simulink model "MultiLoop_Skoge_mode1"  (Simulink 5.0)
settings: Solver=ode1  SolverMode=SingleTasking  StartTime=0.0  StopTime=100  FixedStep=Ts_base  MaxStep=Ts_base  MinStep=1e-6  RelTol=1e-6
PreLoadFcn:
  | Skoge_Mode1_Init
StopFcn:
  | teplot
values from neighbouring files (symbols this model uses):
  Ts_base = 0.0005    [Skoge_Mode1_Init.m]
  Ts_save = 0.01    [Skoge_Mode1_Init.m]
libraries: TElib x17, simulink x8

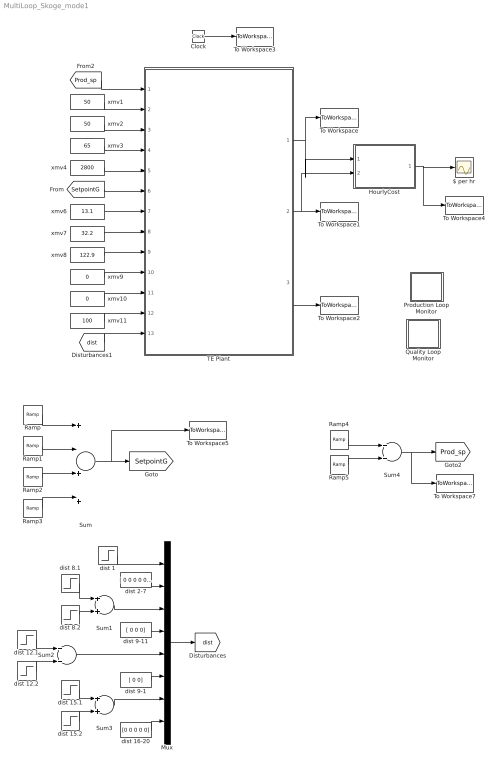
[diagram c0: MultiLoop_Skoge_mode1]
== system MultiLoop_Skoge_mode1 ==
  $ per hr : Scope
  Clock : Clock
  HourlyCost : Subsystem
  Mux : Mux  Inputs=8
  Production Loop Monitor : Subsystem
  Quality Loop Monitor : Subsystem
  Ramp : simulink/Sources/Ramp  slope=-1  start=35  X0=53.8
  Ramp1 : simulink/Sources/Ramp  slope=1  start=45  X0=0
  Ramp2 : simulink/Sources/Ramp  slope=1  start=50  X0=0
  Ramp3 : simulink/Sources/Ramp  slope=-1  start=60  X0=0
  Ramp4 : simulink/Sources/Ramp  slope=.25  start=80  X0=22.89
  Ramp5 : simulink/Sources/Ramp  slope=-.25  start=95  X0=0
  Sum : Sum  Inputs=+|+|+|+  ShowAdditionalParam=on
  Sum{1..4} (4 alike) : Sum
  TE Plant : Subsystem
  To Workspace : ToWorkspace  VariableName=simout  SampleTime=Ts_save  SaveFormat=Array
  To Workspace1 : ToWorkspace  VariableName=xmv  SampleTime=Ts_save  SaveFormat=Array
  To Workspace2 : ToWorkspace  VariableName=idv  SampleTime=Ts_save  SaveFormat=Array
  To Workspace3 : ToWorkspace  VariableName=tout  SampleTime=Ts_save  SaveFormat=Array
  To Workspace4 : ToWorkspace  VariableName=OpCost  SampleTime=Ts_save  SaveFormat=Array
  To Workspace5 : ToWorkspace  VariableName=molG_sp  SampleTime=Ts_save  SaveFormat=Array
  To Workspace7 : ToWorkspace  VariableName=Prod_sp  SampleTime=Ts_save  SaveFormat=Array
  dist 1 : Step  Time=22  Before=1  After=0  SampleTime=0
  dist 12.1 : Step  Time=65  SampleTime=0
  dist 12.2 : Step  Time=70  After=-1  SampleTime=0
  dist 15.1 : Step  Time=65  SampleTime=0
  dist 15.2 : Step  Time=70  After=-1  SampleTime=0
  dist 16-20 : Constant  Value=[0 0 0 0 0]
  dist 2-7 : Constant  Value=[ 0 0 0 0 0 0]
  dist 8.1 : Step  Time=70  SampleTime=0
  dist 8.2 : Step  Time=75  After=-1  SampleTime=0
  dist 9-1 : Constant  Value=[ 0 0]
  dist 9-11 : Constant  Value=[ 0 0 0]
  xmv1 : Constant  Value=50
  xmv10 : Constant  Value=0
  xmv11 : Constant  Value=100
  xmv2 : Constant  Value=50
  xmv3 : Constant  Value=65
  xmv4 : Constant  Value=2800
  xmv6 : Constant  Value=13.1
  xmv7 : Constant  Value=32.2
  xmv8 : Constant  Value=122.9
  xmv9 : Constant  Value=0
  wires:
  TE Plant/1(xmeas) -> To Workspace/1, HourlyCost/1(xmeas)
  xmv1/1 -> TE Plant/2(Strip Level Setpoint)
  xmv2/1 -> TE Plant/3(Sep Level Setpoint)
  xmv3/1 -> TE Plant/4(Reactor Level Setpoint)
  xmv4/1 -> TE Plant/5(Reactor Press Setpoint)
  xmv8/1 -> TE Plant/9(Reactor Temp Setpoint)
  xmv6/1 -> TE Plant/7(%C Setpoint)
  xmv7/1 -> TE Plant/8(Recycle Rate Setpt)
  TE Plant/2(xmv) -> To Workspace1/1, HourlyCost/2(xmv)
  TE Plant/3(idv) -> To Workspace2/1
  Clock/1 -> To Workspace3/1
  HourlyCost/1($ per hr) -> $ per hr/1, To Workspace4/1
  xmv9/1 -> TE Plant/10(Recycle Valve Position)
  xmv10/1 -> TE Plant/11(Steam Valve Position)
  xmv11/1 -> TE Plant/12(Agitator Setting)
  [dist] -> TE Plant/13(Disturbances)
  [SetpointG] -> TE Plant/6(Mole % G Setpoint)
  Ramp/1 -> Sum/1
  Ramp1/1 -> Sum/2
  Ramp2/1 -> Sum/3
  Ramp3/1 -> Sum/4
  Sum/1 -> [SetpointG], To Workspace5/1
  [Prod_sp] -> TE Plant/1(Production Setpoint)
  dist 1/1 -> Mux/1
  dist 2-7/1 -> Mux/2
  dist 8.1/1 -> Sum1/1
  dist 8.2/1 -> Sum1/2
  dist 12.1/1 -> Sum2/1
  dist 12.2/1 -> Sum2/2
  dist 15.1/1 -> Sum3/1
  dist 15.2/1 -> Sum3/2
  Sum1/1 -> Mux/3
  dist 9-11/1 -> Mux/4
  Sum2/1 -> Mux/5
  dist 9-1/1 -> Mux/6
  Sum3/1 -> Mux/7
  dist 16-20/1 -> Mux/8
  Mux/1 -> [dist]
  Ramp4/1 -> Sum4/1
  Ramp5/1 -> Sum4/2
  Sum4/1 -> [Prod_sp], To Workspace7/1

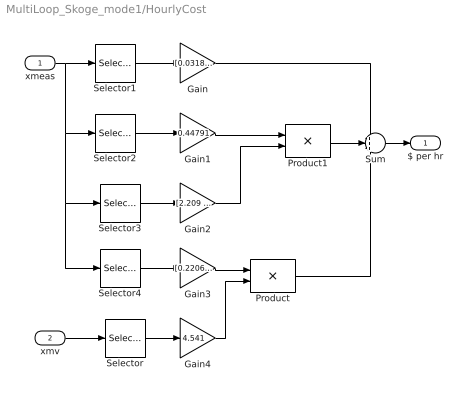
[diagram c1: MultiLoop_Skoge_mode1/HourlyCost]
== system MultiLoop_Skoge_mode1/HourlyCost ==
  xmeas : Inport  PortDimensions=41
  xmv : Inport  Port=2  PortDimensions=12
  Gain : Gain  Gain=[0.0318, 0.0536]  Multiplication=Matrix(K*u)
  Gain1 : Gain  Gain=0.44791
  Gain2 : Gain  Gain=[2.209 6.177 22.06 14.56 17.89 30.44 22.94]  Multiplication=Matrix(K*u)
  Gain3 : Gain  Gain=[0.2206 0.1456 0.1789]  Multiplication=Matrix(K*u)
  Gain4 : Gain  Gain=4.541
  Product : Product
  Product1 : Product
  Selector : Selector  Elements=8  InputPortWidth=12
  Selector1 : Selector  Elements=[19 20]  InputPortWidth=41
  Selector2 : Selector  Elements=[10]  InputPortWidth=41
  Selector3 : Selector  Elements=[29, 31:36]  InputPortWidth=41
  Selector4 : Selector  Elements=[37:39]  InputPortWidth=41
  Sum : Sum  Inputs=+++
  $ per hr : Outport
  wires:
  xmv/1 -> Selector/1
  xmeas/1 -> Selector1/1, Selector2/1, Selector3/1, Selector4/1
  Selector1/1 -> Gain/1
  Selector2/1 -> Gain1/1
  Selector3/1 -> Gain2/1
  Selector4/1 -> Gain3/1
  Selector/1 -> Gain4/1
  Gain3/1 -> Product/1
  Gain4/1 -> Product/2
  Sum/1 -> $ per hr/1
  Product/1 -> Sum/3
  Gain/1 -> Sum/1
  Product1/1 -> Sum/2
  Gain1/1 -> Product1/1
  Gain2/1 -> Product1/2

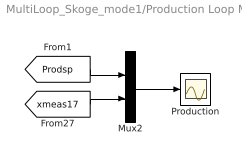
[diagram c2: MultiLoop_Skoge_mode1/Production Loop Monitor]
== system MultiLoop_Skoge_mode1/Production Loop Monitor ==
  Mux2 : Mux  Inputs=2
  Production : Scope
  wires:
  Mux2/1 -> Production/1
  [xmeas17] -> Mux2/2
  [Prodsp] -> Mux2/1

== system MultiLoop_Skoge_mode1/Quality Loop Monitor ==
  Mux2 : Mux  Inputs=2
  Quality : Scope
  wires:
  [PctGsp] -> Mux2/1
  [xmeas40] -> Mux2/2
  Mux2/1 -> Quality/1

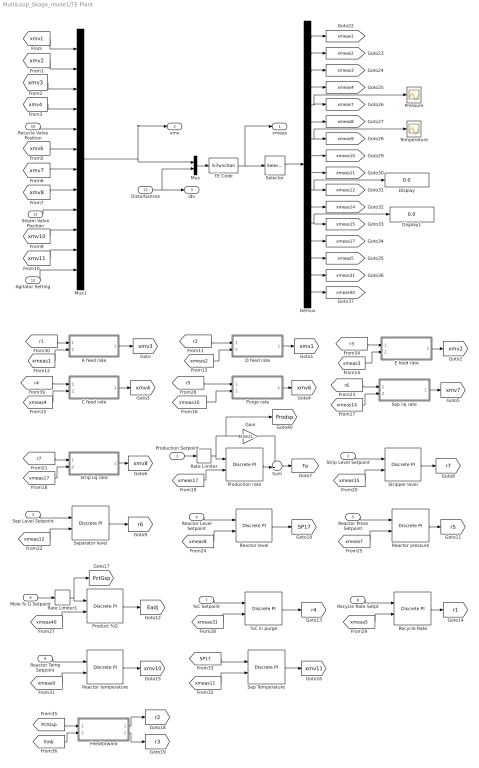
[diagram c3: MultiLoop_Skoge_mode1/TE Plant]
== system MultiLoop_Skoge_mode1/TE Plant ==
  Production Setpoint : Inport
  Strip Level Setpoint : Inport  Port=2
  Sep Level Setpoint : Inport  Port=3
  Reactor Level Setpoint : Inport  Port=4
  Reactor Press Setpoint : Inport  Port=5
  Mole % G Setpoint : Inport  Port=6
  %C Setpoint : Inport  Port=7
  Recycle Rate Setpt : Inport  Port=8
  Reactor Temp Setpoint : Inport  Port=9
  Recycle Valve Position : Inport  Port=10
  Steam Valve Position : Inport  Port=11
  Agitator Setting : Inport  Port=12
  Disturbances : Inport  Port=13
  %C in purge : TElib/Discrete PI  Kc=0.0009  Ti=562/60  Ts=Ts_base  x0=r4_0  Hi=200  Lo=0
  A feed rate : Subsystem
  C feed rate : Subsystem
  D feed rate : Subsystem
  Demux : Demux  Outputs=16
  Display : Display
  Display1 : Display
  E feed rate : Subsystem
  Feedforward : Subsystem
  Gain : Gain  Gain=100/22.89
  Mux : Mux  Inputs=2
  Mux1 : Mux  Inputs=12
  Pressure : Scope
  Product %G : TElib/Discrete PI  Kc=-0.032  Ti=100/60  Ts=Ts_base  x0=Eadj_0  Hi=inf  Lo=-inf
  Production rate : TElib/Discrete PI  Kc=3.2  Ti=120/60  Ts=Ts_base  x0=0  Hi=20  Lo=-20
  Purge rate : Subsystem
  Rate Limiter : RateLimiter  RisingSlewLimit=0.3*22.95/24  FallingSlewLimit=-0.3*22.95/24
  Rate Limiter1 : RateLimiter  RisingSlewLimit=50/24  FallingSlewLimit=-50/24
  Reactor level : TElib/Discrete PI  Kc=0.8  Ti=60/60  Ts=Ts_base  x0=SP17_0  Hi=120  Lo=0
  Reactor pressure : TElib/Discrete PI  Kc=-1e-4  Ti=20/60  Ts=Ts_base  x0=r5_0  Hi=100  Lo=0
  Reactor temperature : TElib/Discrete PI  Kc=-8  Ti=7.5/60  Ts=Ts_base  x0=xmv10_0  Hi=100  Lo=0
  Recycle Rate : TElib/Discrete PI  Kc=0.00125  Ti=120/60  Ts=Ts_base  x0=r1_0  Hi=200  Lo=0
  Selector : Selector  Elements=[1:4, 7:12, 14, 15, 17, 5, 31, 40]  InputPortWidth=41
  Sep Temperature : TElib/Discrete PI  Kc=-4  Ti=15/60  Ts=Ts_base  x0=xmv11_0  Hi=100  Lo=0
  Sep liq rate : Subsystem
  Separator level : TElib/Discrete PI  Kc=-1e-3  Ti=200/60  Ts=Ts_base  x0=r6_0  Hi=100  Lo=0
  Strip liq rate : Subsystem
  Stripper level : TElib/Discrete PI  Kc=-2e-4  Ti=200/60  Ts=Ts_base  x0=r7_0  Hi=100  Lo=0
  Sum : Sum  Inputs=++|
  TE Code : S-Function  FunctionName=temexd  Parameters=[]
  Temperature : Scope
  xmeas : Outport
  xmv : Outport  Port=2
  idv : Outport  Port=3
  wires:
  Mux/1 -> TE Code/1
  Disturbances/1 -> Mux/2, idv/1
  TE Code/1 -> xmeas/1, Selector/1
  [xmv1] -> Mux1/1
  [xmv2] -> Mux1/2
  [xmv3] -> Mux1/3
  [xmv4] -> Mux1/4
  Recycle Valve Position/1 -> Mux1/5
  [xmv6] -> Mux1/6
  [xmv7] -> Mux1/7
  [xmv8] -> Mux1/8
  Steam Valve Position/1 -> Mux1/9
  [xmv10] -> Mux1/10
  [xmv11] -> Mux1/11
  Agitator Setting/1 -> Mux1/12
  A feed rate/1(Valve %) -> [xmv3]
  [xmeas1] -> A feed rate/2(Measured Flow)
  D feed rate/1(Valve %) -> [xmv1]
  [xmeas2] -> D feed rate/2(Measured Flow)
  E feed rate/1(Valve %) -> [xmv2]
  [xmeas3] -> E feed rate/2(Measured Flow)
  C feed rate/1(Valve %) -> [xmv4]
  [xmeas4] -> C feed rate/2(Measured Flow)
  Purge rate/1(Valve %) -> [xmv6]
  [xmeas10] -> Purge rate/2(Measured Flow)
  Sep liq rate/1(Valve %) -> [xmv7]
  [xmeas14] -> Sep liq rate/2(Measured Flow)
  Strip liq rate/1(Valve %) -> [xmv8]
  [xmeas17] -> Strip liq rate/2(Measured Flow)
  [xmeas17] -> Production rate/2
  [xmeas15] -> Stripper level/2
  Strip Level Setpoint/1 -> Stripper level/1
  Stripper level/1 -> [r7]
  [r7] -> Strip liq rate/1(Ratio)
  [xmeas12] -> Separator level/2
  Sep Level Setpoint/1 -> Separator level/1
  Separator level/1 -> [r6]
  [r6] -> Sep liq rate/1(Ratio)
  [xmeas8] -> Reactor level/2
  Reactor Level Setpoint/1 -> Reactor level/1
  Reactor level/1 -> [SP17]
  [xmeas7] -> Reactor pressure/2
  Reactor Press Setpoint/1 -> Reactor pressure/1
  Reactor pressure/1 -> [r5]
  [r5] -> Purge rate/1(Ratio)
  [xmeas40] -> Product %G/2
  Product %G/1 -> [Eadj]
  [xmeas31] -> %C in purge/2
  %C Setpoint/1 -> %C in purge/1
  %C in purge/1 -> [r4]
  [xmeas5] -> Recycle Rate/2
  Recycle Rate Setpt/1 -> Recycle Rate/1
  Recycle Rate/1 -> [r1]
  [r1] -> A feed rate/1(Ratio)
  [xmeas9] -> Reactor temperature/2
  Reactor Temp Setpoint/1 -> Reactor temperature/1
  Reactor temperature/1 -> [xmv10]
  [xmeas11] -> Sep Temperature/2
  [SP17] -> Sep Temperature/1
  Sep Temperature/1 -> [xmv11]
  [r2] -> D feed rate/1(Ratio)
  [r3] -> E feed rate/1(Ratio)
  [PctGsp] -> Feedforward/1(Mole % G SP)
  [Eadj] -> Feedforward/2(Eadj)
  Feedforward/1(r2) -> [r2]
  Feedforward/2(r3) -> [r3]
  Mux1/1 -> Mux/1, xmv/1
  Selector/1 -> Demux/1
  Demux/1 -> [xmeas1]
  Demux/2 -> [xmeas2]
  Demux/3 -> [xmeas3]
  Demux/4 -> [xmeas4]
  Demux/5 -> [xmeas7], Pressure/1
  Demux/6 -> [xmeas8]
  Demux/7 -> [xmeas9], Temperature/1
  Demux/8 -> [xmeas10]
  Demux/9 -> [xmeas11]
  Demux/10 -> [xmeas12], Display/1
  Demux/11 -> [xmeas14]
  Demux/12 -> [xmeas15], Display1/1
  Demux/13 -> [xmeas17]
  Demux/14 -> [xmeas5]
  Demux/15 -> [xmeas31]
  Demux/16 -> [xmeas40]
  [r4] -> C feed rate/1(Ratio)
  Rate Limiter1/1 -> Product %G/1, [PctGsp]
  Mole % G Setpoint/1 -> Rate Limiter1/1
  Rate Limiter/1 -> Production rate/1, Gain/1, [Prodsp]
  Production Setpoint/1 -> Rate Limiter/1
  Sum/1 -> [Fp]
  Production rate/1 -> Sum/2
  Gain/1 -> Sum/1

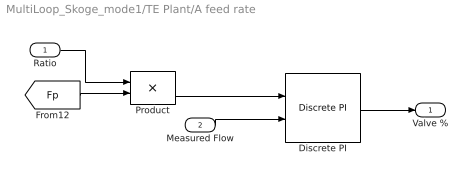
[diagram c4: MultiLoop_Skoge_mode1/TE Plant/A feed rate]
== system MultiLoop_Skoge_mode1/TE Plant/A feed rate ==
  Ratio : Inport
  Measured Flow : Inport  Port=2
  Discrete PI : TElib/Discrete PI  Kc=0.01  Ti=0.001/60  Ts=Ts_base  x0=xmv3_0  Hi=100  Lo=0
  Product : Product
  Valve % : Outport
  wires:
  Discrete PI/1 -> Valve %/1
  Ratio/1 -> Product/1
  [Fp] -> Product/2
  Measured Flow/1 -> Discrete PI/2
  Product/1 -> Discrete PI/1

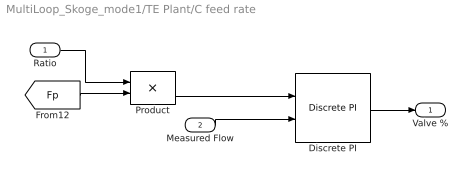
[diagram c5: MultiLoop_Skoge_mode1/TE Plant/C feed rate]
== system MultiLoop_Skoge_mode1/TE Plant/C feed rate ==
  Ratio : Inport
  Measured Flow : Inport  Port=2
  Discrete PI : TElib/Discrete PI  Kc=0.003  Ti=0.001/60  Ts=Ts_base  x0=xmv4_0  Hi=100  Lo=0
  Product : Product
  Valve % : Outport
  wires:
  Product/1 -> Discrete PI/1
  Measured Flow/1 -> Discrete PI/2
  [Fp] -> Product/2
  Ratio/1 -> Product/1
  Discrete PI/1 -> Valve %/1

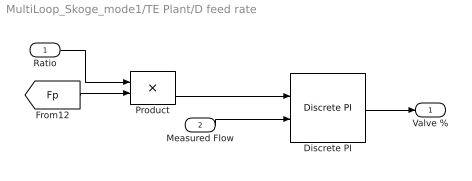
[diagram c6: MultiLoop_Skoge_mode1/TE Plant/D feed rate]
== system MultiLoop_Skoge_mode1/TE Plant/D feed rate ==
  Ratio : Inport
  Measured Flow : Inport  Port=2
  Discrete PI : TElib/Discrete PI  Kc=1.6e-6  Ti=0.001/60  Ts=Ts_base  x0=xmv1_0  Hi=100  Lo=0
  Product : Product
  Valve % : Outport
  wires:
  Product/1 -> Discrete PI/1
  Measured Flow/1 -> Discrete PI/2
  [Fp] -> Product/2
  Ratio/1 -> Product/1
  Discrete PI/1 -> Valve %/1

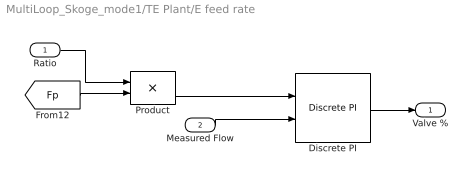
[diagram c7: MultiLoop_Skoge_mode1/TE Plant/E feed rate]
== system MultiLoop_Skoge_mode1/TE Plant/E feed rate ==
  Ratio : Inport
  Measured Flow : Inport  Port=2
  Discrete PI : TElib/Discrete PI  Kc=1.8e-6  Ti=0.001/60  Ts=Ts_base  x0=xmv2_0  Hi=100  Lo=0
  Product : Product
  Valve % : Outport
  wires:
  Product/1 -> Discrete PI/1
  Measured Flow/1 -> Discrete PI/2
  [Fp] -> Product/2
  Ratio/1 -> Product/1
  Discrete PI/1 -> Valve %/1

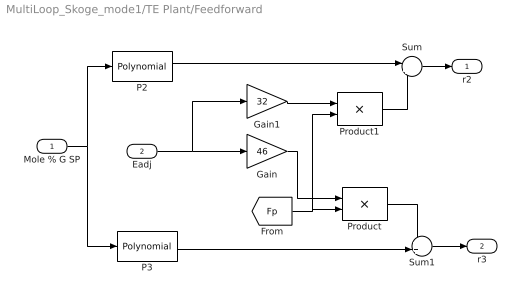
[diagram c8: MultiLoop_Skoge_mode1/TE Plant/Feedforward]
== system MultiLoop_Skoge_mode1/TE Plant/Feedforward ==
  Mole % G SP : Inport
  Eadj : Inport  Port=2
  Gain : Gain  Gain=46
  Gain1 : Gain  Gain=32
  P2 : simulink/Math Operations/Polynomial  coefs="[1.5192e-003  5.9446e-001  2.7690e-001]"
  P3 : simulink/Math Operations/Polynomial  coefs="[-1.1377e-003 -8.0893e-001  9.1060e+001]"
  Product : Product  Inputs=*/
  Product1 : Product  Inputs=*/
  Sum : Sum  Inputs=|+-
  Sum1 : Sum  Inputs=++|
  r2 : Outport
  r3 : Outport  Port=2
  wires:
  Mole % G SP/1 -> P2/1, P3/1
  Sum/1 -> r2/1
  P2/1 -> Sum/1
  Sum1/1 -> r3/1
  P3/1 -> Sum1/2
  Product/1 -> Sum1/1
  [Fp] -> Product/2, Product1/2
  Gain/1 -> Product/1
  Eadj/1 -> Gain/1, Gain1/1
  Product1/1 -> Sum/2
  Gain1/1 -> Product1/1

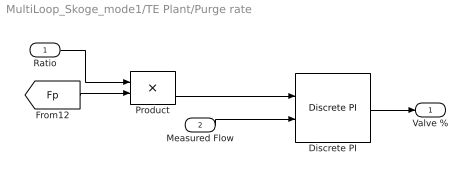
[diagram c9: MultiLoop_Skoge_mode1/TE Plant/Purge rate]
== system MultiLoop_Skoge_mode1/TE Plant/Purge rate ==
  Ratio : Inport
  Measured Flow : Inport  Port=2
  Discrete PI : TElib/Discrete PI  Kc=0.01  Ti=0.001/60  Ts=Ts_base  x0=xmv6_0  Hi=100  Lo=0
  Product : Product
  Valve % : Outport
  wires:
  Discrete PI/1 -> Valve %/1
  Ratio/1 -> Product/1
  [Fp] -> Product/2
  Measured Flow/1 -> Discrete PI/2
  Product/1 -> Discrete PI/1

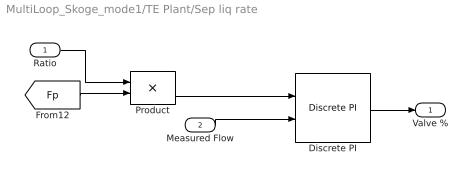
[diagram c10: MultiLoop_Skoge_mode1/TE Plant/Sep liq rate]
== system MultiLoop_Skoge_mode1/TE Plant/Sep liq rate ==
  Ratio : Inport
  Measured Flow : Inport  Port=2
  Discrete PI : TElib/Discrete PI  Kc=4e-4  Ti=0.001/60  Ts=Ts_base  x0=xmv7_0  Hi=100  Lo=0
  Product : Product
  Valve % : Outport
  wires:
  Product/1 -> Discrete PI/1
  Measured Flow/1 -> Discrete PI/2
  [Fp] -> Product/2
  Ratio/1 -> Product/1
  Discrete PI/1 -> Valve %/1

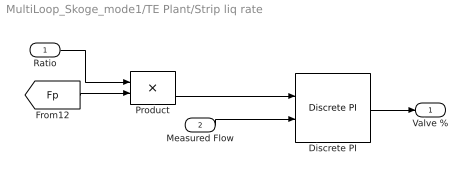
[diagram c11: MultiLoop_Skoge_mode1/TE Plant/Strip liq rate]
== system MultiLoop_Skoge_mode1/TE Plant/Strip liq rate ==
  Ratio : Inport
  Measured Flow : Inport  Port=2
  Discrete PI : TElib/Discrete PI  Kc=4e-4  Ti=0.001/60  Ts=Ts_base  x0=xmv8_0  Hi=100  Lo=0
  Product : Product
  Valve % : Outport
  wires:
  Discrete PI/1 -> Valve %/1
  Ratio/1 -> Product/1
  [Fp] -> Product/2
  Measured Flow/1 -> Discrete PI/2
  Product/1 -> Discrete PI/1
